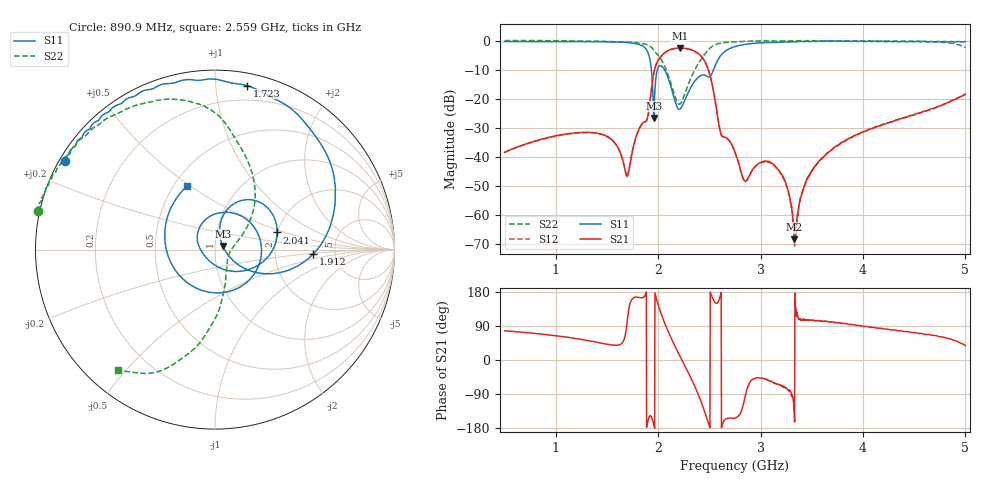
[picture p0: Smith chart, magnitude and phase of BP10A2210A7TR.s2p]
!Agilent Technologies,E8358A,US41080443,A.07.50.56
!Agilent E8358A: A.07.50.56
!Date: Wednesday, July 08, 2015 12:59:15
!Correction: S11(Full 2 Port(1,2))
!S21(Full 2 Port(1,2))
!S12(Full 2 Port(1,2))
!S22(Full 2 Port(1,2))
!S2P File: Measurements: S11, S21, S12, S22:
# Hz S  dB  R 50
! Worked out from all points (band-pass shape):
!   1601 points, 500 MHz to 5 GHz, reference 50 ohm
!   highest |S21| = -2.43 dB at 2.21 GHz (marker M1); lowest = -68.3 dB at 3.329 GHz (marker M2)
!   |S21| within 3 dB of the highest: 2.024 GHz to 2.425 GHz (401.2 MHz wide, 18 % of centre)
!   lowest |S11| = -26.5 dB at 1.957 GHz (marker M3), VSWR 1.10, Z = 54.4 + j2.18 ohm
!   |S11| at or under -10 dB: 1.934 GHz to 1.991 GHz (57.2 MHz wide, 2.91 % of centre); 2.063 GHz to 2.539 GHz (475.4 MHz wide, 20.7 % of centre)
!   |S22| runs from -21.8 to 0.2 dB; largest |S21 - S12| = 0.011
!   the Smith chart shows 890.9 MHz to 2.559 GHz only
!   S11 on the Smith chart (normalised r, x): 890.9 MHz: 0.02, +0.27; 1.723 GHz: 0.09, +1.21; 1.912 GHz: 3.40, -0.25; 2.041 GHz: 2.00, +0.44; 2.559 GHz: 0.58, +0.48
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5e8  -0.19 164.2  -38.34 77.1  -38.45 77.2  0.11 174.7
8.909375e8  -0.27 149.3  -33.56 67.4  -33.66 67.4  0.08 167.7
1.250938e9  -0.22 130.4  -31.48 54.3  -31.59 54.3  -0.03 158.5
1.723438e9  -0.62 78.9  -42.44 147.6  -42.55 147.7  -0.46 131.7
1.911875e9  -5.24 -2.7  -22.75 -149.9  -22.88 -149.9  -1.64 98.2
1.956875e9  -26.53 25.0  -11.05 -170.8  -11.17 -171.0  -3.17 84.4
2.001875e9  -8.98 49.8  -6.49 143.5  -6.57 143.5  -5.03 73.3
2.04125e9  -8.88 15.4  -4.72 112.7  -4.83 112.8  -7.10 60.6
2.117188e9  -14.92 -42.6  -2.95 63.2  -3.05 63.2  -13.80 33.2
2.21e9  -23.55 -144.8  -2.43 11.5  -2.54 11.5  -21.74 -24.7
2.3675e9  -13.42 76.3  -3.74 -75.8  -3.83 -75.7  -9.27 -86.7
2.485625e9  -12.38 -92.6  -9.48 -162.4  -9.61 -162.3  -3.24 -110.5
2.55875e9  -8.27 114.0  -21.12 150.7  -21.22 151.0  -1.29 -128.7
2.654375e9  -3.52 21.1  -33.10 -156.6  -33.20 -157.0  -0.50 -146.3
2.75e9  -1.95 -24.4  -38.29 -153.4  -38.40 -152.9  -0.34 -156.6
2.848438e9  -1.18 -52.2  -48.23 -97.0  -48.33 -96.9  -0.10 -164.3
3.174688e9  -0.42 -97.8  -44.54 -64.2  -44.45 -65.3  0.05 -179.6
3.329375e9  -0.30 -110.5  -68.32 -140.2  -68.29 -149.2  0.08 174.8
3.500938e9  -0.12 -121.9  -44.50 104.4  -44.80 103.7  0.03 171.2
4.251875e9  -0.13 -165.8  -28.04 80.7  -28.14 80.8  -0.03 153.8
4.735625e9  -0.19 -178.5  -22.49 62.2  -22.61 62.2  -0.32 132.9
5e9  -0.21 -178.0  -18.27 37.8  -18.39 37.6  -2.32 89.1
